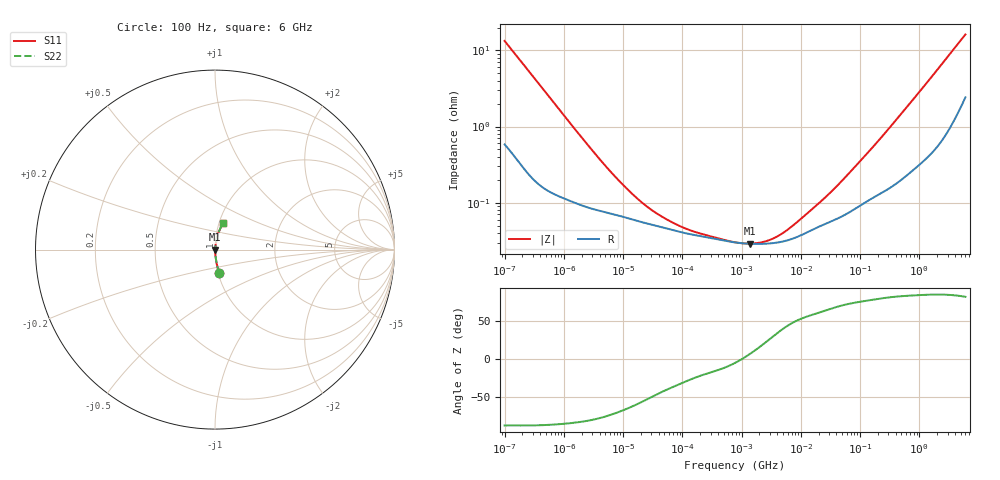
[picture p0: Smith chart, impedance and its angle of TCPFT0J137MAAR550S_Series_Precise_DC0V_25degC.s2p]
! TCPFT0J137MAAR550S Polymer Tantalum Capacitor Sparameter Model
! Model Generated by Samsung Electro-Mechanics
! Samsung Sparameter Version 5.0
! Date : Oct-21-2025
! Products : Polymer Tantalum Capacitor
! Characteristics :
!  Nominal Capacitance = 135uF
!  Capacitance Tolerance = +/-20%
!  ESR = 55 mohm max at 100kHz
!  Rated Voltage = 6.3Vdc
!  Size = 1206(unit:inch), 3216(unit:mm)
!  Length = 3.20+/-0.20mm
!  Width = 1.60+/-0.20mm
!  Thickness = 0.90+/-0.10mm
!  Lineup = Conductive Polymer Type
!  Feature = PFT
!  Measurement Temperature : 25degC.
!  DC bias Value = 0V
!  Frequency : 100Hz ~ 6GHz
! External Node Assignments :
!  1  o---||---o  2
# MHz S RI R 50.0
! Freq.  Real(S11)  Im(S11)  Real(S12)  Im(S12)  Real(S21)  Im(S21)  Real(S22)  Im(S22)
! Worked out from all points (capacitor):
!   300 points, 100 Hz to 6 GHz, reference 50 ohm
!   read as one part in series: C = 118 uF near 106.2 Hz
!   lowest |Z| = 29.1 mohm at 1.368 MHz (marker M1)
!   series resonance near 1.03 MHz, so ESL is about 200 pH
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0.0001  0.0229 -0.1295  0.9771 0.1295  0.9771 0.1295  0.0229 -0.1295
0.0001714451  0.00959 -0.078  0.9904 0.078  0.9904 0.078  0.00959 -0.078
0.0003313429  0.0036 -0.0412  0.9964 0.0412  0.9964 0.0412  0.0036 -0.0412
0.001998454  0.000972 -0.00712  0.999 0.00712  0.999 0.00712  0.000972 -0.00712
0.005210943  0.000753 -0.00286  0.9992 0.00286  0.9992 0.00286  0.000753 -0.00286
0.01069259  0.000644 -0.00149  0.9994 0.00149  0.9994 0.00149  0.000644 -0.00149
0.02194065  0.000549 -0.000801  0.9995 0.000801  0.9995 0.000801  0.000549 -0.000801
0.03993819  0.000488 -0.000495  0.9995 0.000495  0.9995 0.000495  0.000488 -0.000495
0.0726988  0.000432 -0.000317  0.9996 0.000317  0.9996 0.000317  0.000432 -0.000317
0.1323324  0.000387 -0.000203  0.9996 0.000203  0.9996 0.000203  0.000387 -0.000203
0.7981464  0.0003 -2.56e-05  0.9997 2.56e-05  0.9997 2.56e-05  0.0003 -2.56e-05
1.368383  0.000289 3.1e-05  0.9997 -3.1e-05  0.9997 -3.1e-05  0.000289 3.1e-05
2.346024  0.000288 0.000102  0.9997 -0.000102  0.9997 -0.000102  0.000288 0.000102
4.022142  0.0003 0.000201  0.9997 -0.000201  0.9997 -0.000201  0.0003 0.000201
6.895764  0.000332 0.000348  0.9997 -0.000348  0.9997 -0.000348  0.000332 0.000348
15.95059  0.000444 0.000711  0.9996 -0.000711  0.9996 -0.000711  0.000444 0.000711
29.03458  0.000548 0.00115  0.9995 -0.00115  0.9995 -0.00115  0.000548 0.00115
49.77836  0.000666 0.00183  0.9993 -0.00183  0.9993 -0.00183  0.000666 0.00183
318.7652  0.00165 0.00961  0.9983 -0.00961  0.9983 -0.00961  0.00165 0.00961
1810.813  0.00737 0.0494  0.9926 -0.0494  0.9926 -0.0494  0.00737 0.0494
3296.191  0.0173 0.0874  0.9827 -0.0874  0.9827 -0.0874  0.0173 0.0874
6000  0.047 0.1492  0.953 -0.1492  0.953 -0.1492  0.047 0.1492
